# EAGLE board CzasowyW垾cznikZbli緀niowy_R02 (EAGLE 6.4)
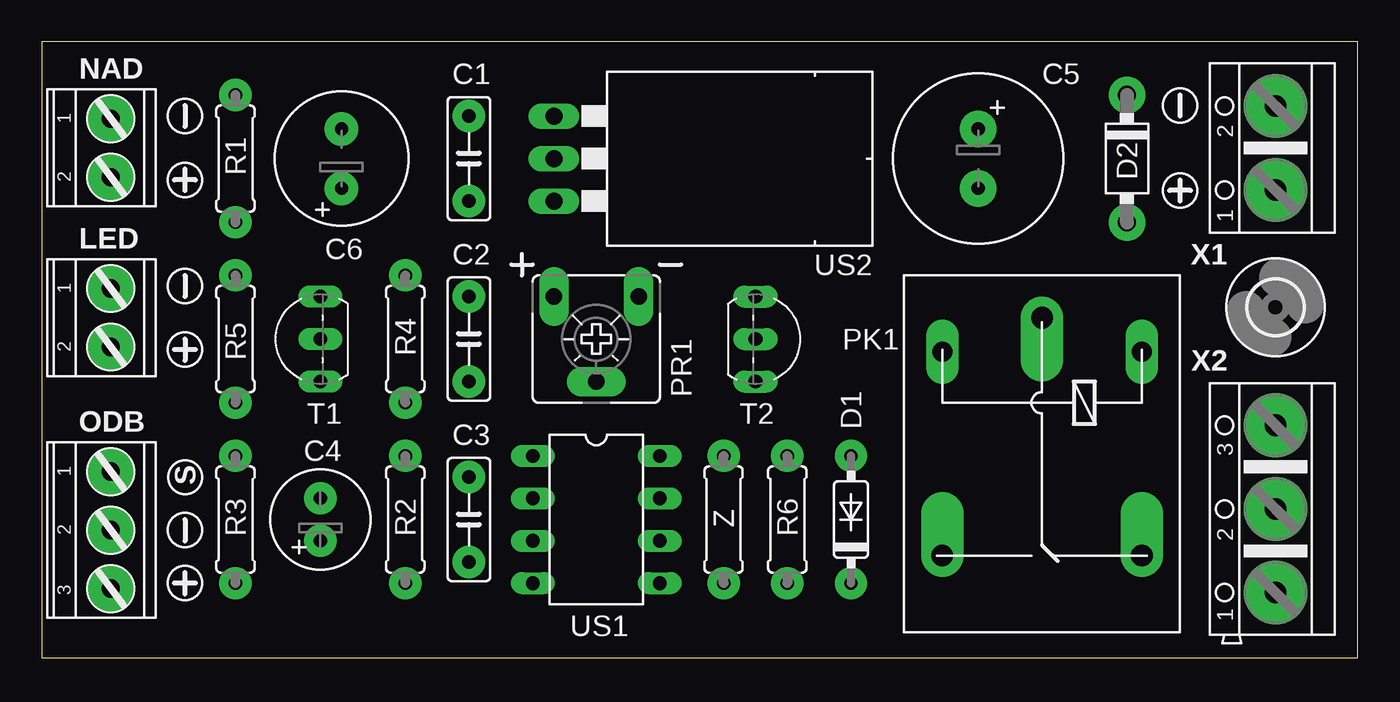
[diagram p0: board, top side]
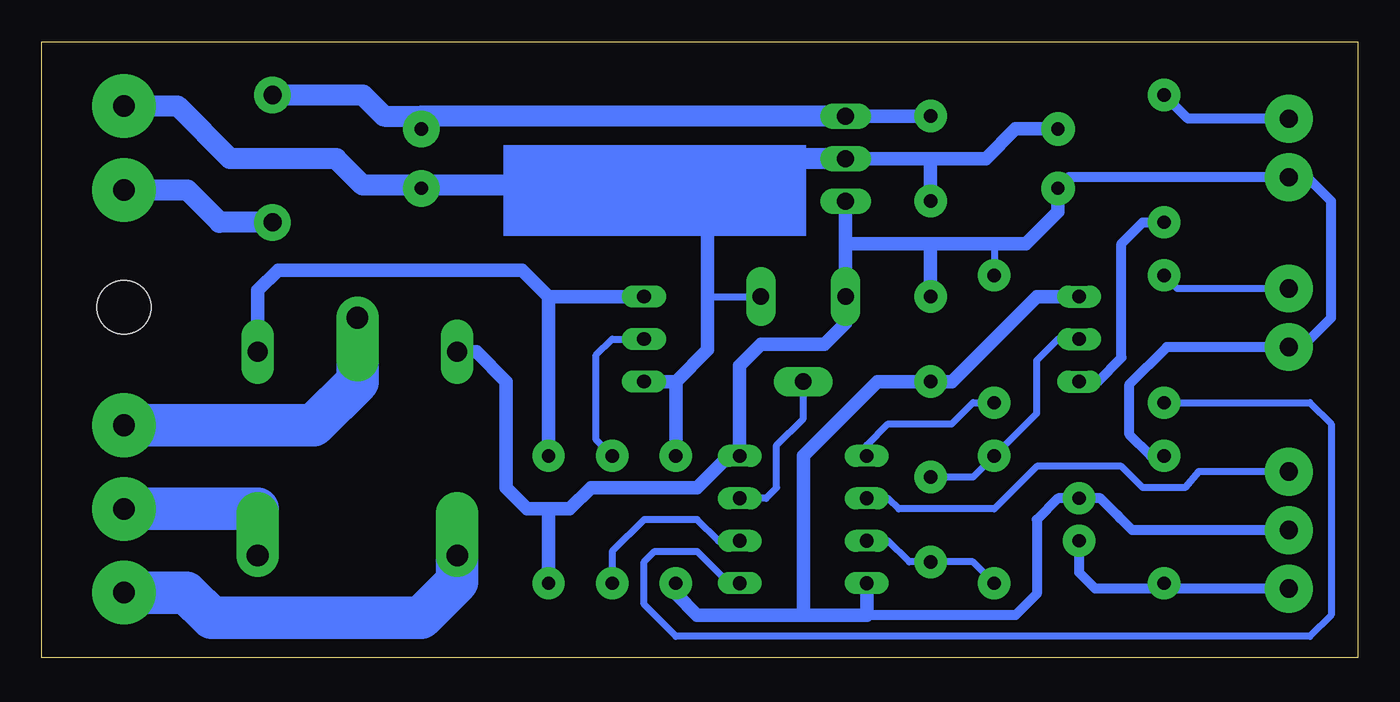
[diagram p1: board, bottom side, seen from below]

Size 78.74 x 36.83 mm. Coordinates in mm from the lower left corner, seen from the top.
Outline: 0,0 78.74,0 78.74,36.83 0,36.83 0,0
Copper layers (1*16): Top 0.035mm / dielectric 1.5mm / Bottom 0.035mm
Design rules "AVT": minimum track width 16mil, minimum drill 19mil, track to track 10mil, track to pad 10mil, pad to pad 10mil, via to via 10mil, smd to smd 10mil, copper to edge 20mil, drill to drill 10mil, minimum pad ring 10mil, minimum via ring 10mil, stop-mask expansion 4mil, vias tented up to drill 0mil, thermal gap 10mil

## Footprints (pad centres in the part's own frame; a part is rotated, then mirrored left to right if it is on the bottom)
C050-025X075 = drill 0.8 pad 1.93: 1 -2.54,0; 2 2.54,0
E2,5-6 = drill 0.8 pad 1.93: + -1.27,0; - 1.27,0
E3,5-10 = drill 0.8 pad 2.184: + -1.778,0; - 1.778,0
E3,5-8 = drill 0.8 pad 2: + -1.778,0; - 1.778,0
DO35-7 = drill 0.8 pad 1.93: A 3.81,0; C -3.81,0
DO41-7.6 = drill 1.1 pad 2.184: A 3.81,0; C -3.81,0
3,2_SMALL = hole 3.2: 0,0
AK550/2 = drill 1.1 pad 2.857: 1 -1.75,0; 2 1.75,0
AK550/3 = drill 1.1 pad 2.857: 1 -3.5,0; 2 0,0; 3 3.5,0
G5LE = drill 1.2 pad 1.93 long: 1 -7.493,-5.969; 2 -7.493,5.969 | drill 1.3 pad 2.54 offset: O 4.699,5.969; P -9.525,0; S 4.699,-5.969
CA6V = drill 1 pad 1.778 long: A -2.54,-2.54; E 2.54,-2.54; S 0,2.54
0207/7 = drill 0.8 pad 1.93: 1 -3.81,0; 2 3.81,0
TO92-EBC = drill 0.813 long: B 0,-1.27; C -2.54,-1.27; E 2.54,-1.27
DIL08 = drill 0.813 long: 1 -3.81,-3.81; 2 -1.27,-3.81; 3 1.27,-3.81; 4 3.81,-3.81; 5 3.81,3.81; 6 1.27,3.81; 7 -1.27,3.81; 8 -3.81,3.81
78XXL_H = drill 1.016 long: GND 0,-3.81; IN -2.54,-3.81; OUT 2.54,-3.81
AK500/2 = drill 1.3 pad 3.81: 1 -2.515,0; 2 2.515,0
AK500/3 = drill 1.3 pad 3.81: 1 -5.004,0; 2 0,0; 3 5.004,0

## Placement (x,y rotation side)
C1  100n  [C050-025X075]  25.56,29.84 90 top
C2  100n  [C050-025X075]  25.56,19.05 90 top
C3  1n  [C050-025X075]  25.56,8.26 90 top
C4  10u  [E2,5-6]  16.67,8.26 90 top
C5  1000u  [E3,5-10]  56.04,29.84 270 top
C6  100u  [E3,5-8]  17.94,29.84 90 top
D1  1N4148DO35-7  [DO35-7]  48.42,8.26 90 top
D2  1N40047.62  [DO41-7.6]  64.93,29.84 270 top
H1  MOUNT-HOLE3,2_SMALL  [3,2_SMALL]  73.82,20.95 0 top
LED  [AK550/2]  4.13,20.32 270 top
NAD  [AK550/2]  4.13,30.48 270 top
ODB  [AK550/3]  4.13,7.62 270 top
PK1  G5L_5V  [G5LE]  59.85,10.79 270 top
PR1  200k  [CA6V]  33.18,19.05 180 top
R1  390  [0207/7]  11.59,29.84 90 top
R2  10k  [0207/7]  21.75,8.26 270 top
R3  390  [0207/7]  11.59,8.26 90 top
R4  10k  [0207/7]  21.75,19.05 90 top
R5  390  [0207/7]  11.59,19.05 270 top
R6  4,7k  [0207/7]  44.61,8.26 270 top
T1  BC548  [TO92-EBC]  15.4,19.05 90 top
T2  BC548  [TO92-EBC]  43.97,19.05 270 top
U$2  +  [+]  68.1,27.94 90 top
U$3  -  [-]  68.1,33.02 90 top
U$4  +  [+]  8.57,28.57 0 top
U$5  -  [-]  8.57,32.38 90 top
U$6  +  [+]  8.57,18.41 90 top
U$7  -  [-]  8.57,22.23 90 top
U$8  +  [+]  8.57,4.45 0 top
U$9  -  [-]  8.57,7.62 90 top
US1  TINY13-20PU  [DIL08]  33.18,8.26 270 top
US2  7805  [78XXL_H]  34.45,29.84 270 top
X1  ZAS  [AK500/2]  73.82,30.48 90 top
X2  NC COM NO  [AK500/3]  73.82,8.89 90 top
Z  0  [0207/7]  40.8,8.26 90 top

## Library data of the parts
C1-C6 R1-R6 Z = rcl
D1 D2 = diode
H1 = holes
LED NAD ODB = con-ptr500+
PK1 = relay; OC_FARNELL: unknown; OC_NEWARK: unknown
PR1 = pot
T1 T2 = transistor-npn
U$2-U$9 = symbole
US1 = atmel; MPN: ATTINY13-20PU; OC_FARNELL: 9171550; OC_NEWARK: 96K6521
US2 = v-reg
X1 X2 = con-ptr500; OC_FARNELL: unknown; OC_NEWARK: unknown

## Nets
+5V: C2.2 C6.+ D1.C LED.2 NAD.2 PK1.1 PR1.E R3.2 R4.2 US1.8 US2.OUT
GND: C1.1 C5.- C6.- PR1.A T2.E US2.GND X1.2 Z.2
LED: R5.2 US1.5
N$1: D1.A PK1.2 T2.C
N$2: C2.1 C4.- ODB.2 T1.E US1.4 Z.1
N$3: R6.1 T2.B
N$4: PK1.S X2.1
N$5: PK1.P X2.3
N$6: PK1.O X2.2
N$7: NAD.1 R1.2
N$8: R1.1 T1.C
N$9: D2.A X1.1
N$12: C1.2 C5.+ D2.C US2.IN
N$14: C3.2 R2.1 T1.B
N$19: C4.+ ODB.3 R3.1
N$22: LED.1 R5.1
PK: R6.2 US1.6
R_IR: ODB.1 US1.2
RES: R4.1 US1.1
T_IR: C3.1 R2.2 US1.3
TIME: PR1.S US1.7

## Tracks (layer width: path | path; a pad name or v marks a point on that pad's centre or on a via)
+5V
  Bottom 0.406: 21.75,24.77 R4.2
  Bottom 0.61: C6.+ 17.28,28.73 NAD.2 3.01,28.73 1.59,27.3 1.59,20.32 3.34,18.57 LED.2 11.43,18.57 13.65,16.35 13.65,13.34 12.38,12.06 R3.2
  Bottom 0.813: 48.42,8.89 47.15,8.89 45.88,10.16 39.53,10.16 37.62,12.06 US1.8 36.99,17.46 35.72,18.73 31.91,18.73 30.64,20 PR1.E 30.64,24.77 | 30.64,24.77 US2.OUT | C6.+ 17.94,26.67 19.84,24.77 21.75,24.77 25.56,24.77 | 25.56,24.77 30.64,24.77 | 25.56,24.77 C2.2 | D1.C 48.42,8.89 | 48.42,8.89 49.69,8.89 50.96,10.16 50.96,16.51 52.74,18.29 PK1.1
GND
  Bottom 0.406: 38.89,21.59 PR1.A
  Bottom 0.813: 40.8,16.51 38.89,18.41 38.89,21.59 38.89,29.84 | 40.8,16.51 T2.E | 25.56,29.84 US2.GND | 25.56,29.84 C1.1 | 40.8,16.51 Z.2 | 25.56,29.84 22.26,29.84 20.48,31.62 C6.-
  Bottom 1.27: US2.GND 38.89,29.84 48.42,29.84 50.01,28.26 56.04,28.26 | 56.04,28.26 59.53,28.26 61.12,29.84 67.47,29.84 70.62,32.99 X1.2 | 56.04,28.26 C5.-
LED
  Bottom 0.406: R5.2 2.86,15.24 1.59,13.97 1.59,2.54 2.86,1.27 40.8,1.27 42.7,3.17 42.7,5.71 42.07,6.35 39.53,6.35 37.62,4.45 US1.5
N$1
  Bottom 0.813: T2.C 48.42,21.59 | 48.42,21.59 D1.A | PK1.2 65.82,21.97 64.61,23.18 50.01,23.18 48.42,21.59
N$2
  Bottom 0.61: 14.13,8.26 14.45,8.57 | 14.45,8.57 15.4,9.53 C4.- 17.94,9.53 19.21,8.26 19.21,3.81 20.48,2.54 29.37,2.54 | 40.8,3.81 40.8,4.13 | ODB.2 13.49,7.62 14.45,8.57
  Bottom 0.813: US1.4 29.37,2.54 33.18,2.54 | 33.18,2.54 39.53,2.54 40.8,3.81 | 40.8,4.13 Z.1 | T1.E 19.21,21.59 24.29,16.51 C2.1 28.73,16.51 33.18,12.06 33.18,2.54
N$3
  Bottom 0.406: T2.B 44.61,19.05 45.56,18.1 45.56,13.02 R6.1
N$4
  Bottom 2.54: X2.1 70.08,3.89 68.58,2.38 56.04,2.38 53.88,4.54 PK1.S
N$5
  Bottom 2.54: X2.3 62.46,13.89 59.85,16.51 PK1.P
N$6
  Bottom 2.54: X2.2 65.82,8.89 PK1.O
N$7
  Bottom 0.61: NAD.1 10.16,32.23 R1.2
N$8
  Bottom 0.61: T1.C 15.56,16.51 14.13,17.94 14.13,24.77 12.86,26.04 R1.1
N$9
  Bottom 1.27: D2.A 68.1,26.04 70.03,27.96 X1.1
N$12
  Bottom 0.813: C1.2 US2.IN
  Bottom 1.27: US2.IN 56.04,32.38 | 56.04,32.38 C5.+ | D2.C 59.53,33.66 58.26,32.38 56.04,32.38
N$14
  Bottom 0.406: C3.2 23.02,10.79 R2.1 19.21,14.61 19.21,17.78 17.94,19.05 T1.B
N$19
  Bottom 0.61: ODB.3 11.59,4.12 | 11.59,4.12 15.71,4.12 16.67,5.08 C4.+ | R3.1 11.59,4.12
N$22
  Bottom 0.406: LED.1 10.8,22.07 R5.1
PK
  Bottom 0.406: US1.6 38.26,6.99 39.53,8.26 42.7,8.26 44.61,6.35 R6.2
R_IR
  Bottom 0.406: US1.2 28.1,9.53 27.46,8.89 21.75,8.89 19.21,11.43 14.13,11.43 12.86,10.16 10.32,10.16 9.52,11.12 ODB.1
RES
  Bottom 0.406: US1.1 29.37,12.7 28.1,13.97 24.29,13.97 23.02,15.24 R4.1
T_IR
  Bottom 0.406: R2.2 23.02,5.71 C3.1 26.83,5.71 28.1,6.99 US1.3
TIME
  Bottom 0.406: US1.7 35.4,9.53 34.77,10.16 34.77,12.7 33.18,14.29 PR1.S
(copper drawn outside any net)
  shapes: Bottom area x1

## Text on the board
tPlace: S
bStop: ZAS | COM NC NO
